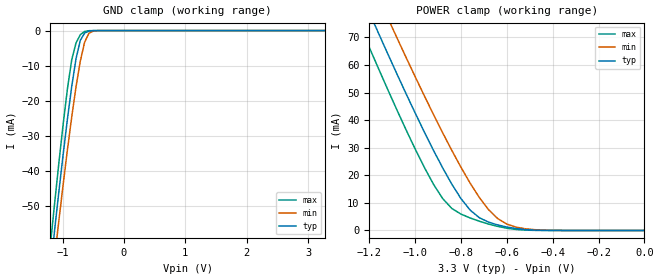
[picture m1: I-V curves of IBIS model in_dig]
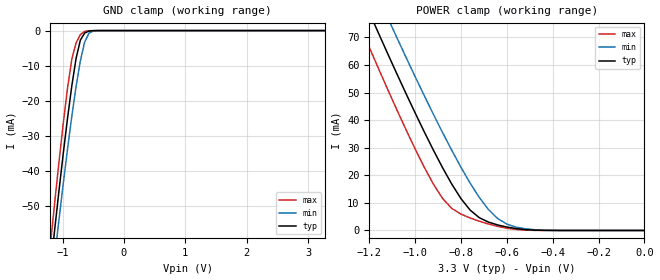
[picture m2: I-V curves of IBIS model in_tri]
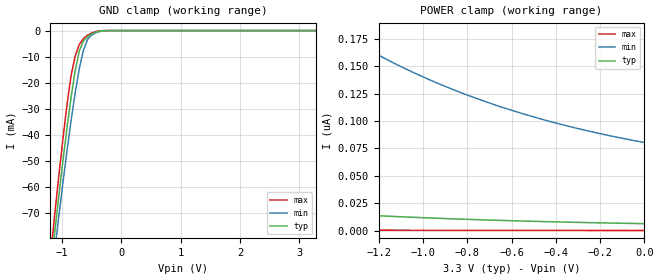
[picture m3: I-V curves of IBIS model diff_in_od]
| Integrated Devices Technolgy, Inc
[Ibis Ver]   4.1
[File Name]   9zxl1930d.ibs
[File Rev]   1.0
[Date]   Tuesday, January 30, 2018
[Source]   Integrated Devices Technolgy, Inc.
[Notes]   Rev 1.0 created by EvK
[Disclaimer] Integrated Device Technology, Inc. ("IDT") hereby grants the
   user of this IBIS model a non-exclusive, nontransferable
   license to use this IBIS model under the following terms. The
   user is granted this license only to use the IBIS model and is
   not granted rights to sell, copy (except as needed to run the
   IBIS model), rent, lease or sub-license the IBIS model in
   whole or in part, or in modified form to anyone. The User may
   modify the IBIS model to suit its specific applications, but
   rights to derivative works and such modifications shall belong
   to IDT. This IBIS model is provided on an AS IS" basis and IDT
   makes absolutely no warranty with respect to the information
   contained herein. IDT DISCLAIMS AND CUSTOMER WAIVES ALL
   WARRANTIES, EXPRESS AND IMPLIED, INCLUDING WARRANTIES OF
   MERCHANTABILITY AND FITNESS FOR A PARTICULAR PURPOSE. THE
   ENTIRE RISK AS TO QUALITY AND PERFORMANCE IS WITH THE USER
   ACCORDINGLY, IN NO EVENT SHALL IDT BE LIABLE FOR ANY DIRECT OR
   INDIRECT DAMAGES, WHETHER IN CONTRACT OR TORT, INCLUDING ANY
   LOST PROFITS OR OTHER INCIDENTAL, CONSEQUENTIAL, EXEMPLARY, OR
   PUNITIVE DAMAGES ARISING OUT OF THE USE OR APPLICATION OF THE
   IBIS model. Further, IDT reserves the right to make changes
   without notice to any product herein to improve reliability,
   function, or design. IDT does not convey any license under
   patent rights or any other intellectual property rights,
   including those of third parties. IDT is not obligated to
   provide maintenance or support for the licensed IBIS model.
   (C) Copyright Integrated Device Technology, Inc. 2016 All
   rights reserved
|   COMPONENT: ICS9zxl1930d
[Component]   ICS9zxl1930d
[Manufacturer]   Integrated Device Technology, Inc.
[Package]
| variable   typ   min   max
R_pkg   81.10m   62.20m   100.00m
L_pkg   6.70nH   4.90nH   8.50nH
C_pkg   0.53pF   0.21pF   0.85pF
[Pin]   signal_name   model_name   R_pin   L_pin   C_pin
1   VDDA   POWER
2   GNDA   GND
3   100M_133M#   in_dig
4   HBW_BYP_LBW#  in_tri
5   CKPWRGD_PD#   in_dig
6   GND   GND
7   VDDR   POWER
8   DIF_IN   diff_in_od
9   DIF_IN#   diff_in_od
10   SADR0_TRI   in_tri_od
11   SMBDAT   sda_od
12   SMBCLK   scl_od
13   SADR1_TRI   in_tri_od
14   FBOUT_NC#   NC
15   FBOUT_NC   NC
16   GND   GND
17   DIF_0   diff_out
18   DIF_0#   diff_out
19   DIF_1   diff_out
20   DIF_1#   diff_out
21   VDDIO   POWER
22   GND   GND
23   DIF_2   diff_out
24   DIF_2#   diff_out
25   DIF_3   diff_out
26   DIF_3#   diff_out
27   GND   GND
28   VDD   POWER
29   DIF_4   diff_out
30   DIF_4#   diff_out
31   DIF_5   diff_out
32   DIF_5#   diff_out
33   VDDIO   POWER
34   GND   GND
35   DIF_6   diff_out
36   DIF_6#   diff_out
37   DIF_7   diff_out
38   DIF_7#   diff_out
39   GND   GND
40   VDDIO   POWER
41   DIF_8   diff_out
42   DIF_8#   diff_out
43   DIF_9   diff_out
44   DIF_9#   diff_out
45   VDD   POWER
46   GND   GND
47   DIF_10   diff_out
48   DIF_10#   diff_out
49   DIF_11   diff_out
50   DIF_11#   diff_out
51   GND   GND
52   VDDIO   POWER
53   DIF_12   diff_out
54   DIF_12#   diff_out
55   DIF_13   diff_out
56   DIF_13#   diff_out
57   VDDIO   POWER
58   GND   GND
59   DIF_14   diff_out
60   DIF_14#   diff_out
61   DIF_15   diff_out
62   DIF_15#   diff_out
63   GND   GND
64   VDD   POWER
65   DIF_16   diff_out
66   DIF_16#   diff_out
67   DIF_17   diff_out
68   DIF_17#   diff_out
69   VDDIO   POWER
70   GND   GND
71   DIF_18   diff_out
72   DIF_18#   diff_out
73   EPAD   GND
[Diff Pin]   inv_pin   vdiff   tdelay_typ
8   9   NA   NA
15   14   NA   NA
17   18   NA   NA
19   20   NA   NA
23   24   NA   NA
25   26   NA   NA
29   30   NA   NA
31   32   NA   NA
35   36   NA   NA
37   38   NA   NA
41   42   NA   NA
43   44   NA   NA
47   48   NA   NA
49   50   NA   NA
53   54   NA   NA
55   56   NA   NA
59   60   NA   NA
61   62   NA   NA
65   66   NA   NA
67   68   NA   NA
71   72   NA   NA
[Model Selector] diff_out
clk_out   HCSL Diff output enabled
hcsl_hiz   HCSL Diff output disabled to Hi-Z
| Models and submodels in the file (8): in_dig (Input), in_tri (Input), diff_in_od (Input), in_tri_od (Input), sda_od (I/O_open_drain), scl_od (Input), hcsl_hiz (Input), clk_out (Output)
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|   Model in_dig
[Model]  in_dig
Model_type Input
Polarity   Non-Inverting
Vinl =   0.8000V
Vinh =   2.0000V
C_comp   2.1000pF   2.1000pF   2.1000pF
[Temperature Range]   25.0000   85.0000   -40.0000
[Voltage Range]   3.3000V   3.1350V   3.4650V
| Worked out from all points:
|   GND clamp passes 1 mA (typ) near -0.65 V on its own axis
|   POWER clamp passes 1 mA (typ) near -0.58 V on its own axis
[GND_clamp]
|Voltage   I(typ)   I(min)   I(max)
-3.3V     -444.4mA   -436.3mA   -455.2mA
-1.2V     -68.37mA   -75.7mA    -61.37mA
-1.13V    -56.99mA   -64.8mA    -49.35mA
-1.06V    -45.92mA   -54.16mA   -37.72mA
-920mV    -25.14mA   -33.91mA   -16.51mA
-850mV    -15.84mA   -24.53mA   -8.255mA
-780mV    -7.95mA    -15.96mA   -3.499mA
-710mV    -2.728mA   -8.626mA   -1.156mA
-640mV    -697.7uA   -3.286mA   -240.6uA
-570mV    -146.6uA   -751uA     -34.01uA
-430mV    -3.844uA   -23.08uA   -279.3nA
3.28V     213.4pA    44.16nA    205.9pA
[POWER_clamp]
|Voltage   I(typ)   I(min)   I(max)
-3.28V    509.3mA    515.8mA    504.9mA
-1.24V    86.61mA    99.33mA    74.1mA
-1.16V    71.55mA    84.5mA     58.72mA
-1.12V    64.14mA    77.19mA    51.18mA
-1.08V    56.84mA    69.96mA    43.78mA
-960mV    35.71mA    48.84mA    22.88mA
-880mV    22.69mA    35.43mA    11.57mA
-840mV    16.77mA    29.02mA    7.979mA
-760mV    7.367mA    17.14mA    4.53mA
-640mV    2.005mA    4.321mA    1.477mA
-480mV    131.2uA    293.3uA    37.64uA
0V        220.8pA    394.5pA    228.5pA
|   Model in_tri
[Model]  in_tri
Model_type Input
Polarity   Non-Inverting
Vinl =   0.8000V
Vinh =   2.0000V
C_comp   2.1400pF   2.1400pF   2.1400pF
[Temperature Range]   25.0000   85.0000   -40.0000
[Voltage Range]   3.3000V   3.1350V   3.4650V
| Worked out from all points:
|   GND clamp passes 1 mA (typ) near -0.65 V on its own axis
|   POWER clamp passes 1 mA (typ) near -0.58 V on its own axis
[GND_clamp]
|Voltage   I(typ)   I(min)   I(max)
-3.3V     -444.4mA   -436.3mA   -455.2mA
-1.2V     -68.37mA   -75.7mA    -61.37mA
-1.13V    -56.99mA   -64.8mA    -49.35mA
-1.06V    -45.92mA   -54.16mA   -37.72mA
-920mV    -25.14mA   -33.91mA   -16.51mA
-850mV    -15.84mA   -24.53mA   -8.255mA
-780mV    -7.95mA    -15.96mA   -3.499mA
-710mV    -2.728mA   -8.625mA   -1.156mA
-640mV    -697.7uA   -3.286mA   -240.6uA
-570mV    -146.6uA   -751uA     -34.01uA
-430mV    -3.844uA   -23.08uA   -279.3nA
3.28V     213.4pA    44.16nA    205.9pA
[POWER_clamp]
|Voltage   I(typ)   I(min)   I(max)
-3.28V    509.3mA    515.8mA    504.9mA
-1.24V    86.61mA    99.33mA    74.1mA
-1.16V    71.55mA    84.5mA     58.72mA
-1.12V    64.14mA    77.19mA    51.18mA
-1.08V    56.84mA    69.96mA    43.78mA
-960mV    35.71mA    48.84mA    22.88mA
-880mV    22.69mA    35.43mA    11.57mA
-840mV    16.77mA    29.02mA    7.979mA
-760mV    7.367mA    17.14mA    4.53mA
-640mV    2.005mA    4.321mA    1.477mA
-480mV    131.2uA    293.3uA    37.64uA
0V        220.8pA    394.5pA    228.4pA
|   Model diff_in_od
[Model]  diff_in_od
Model_type Input
Polarity   Non-Inverting
Vinl =   0.3000V
Vinh =   0.5000V
C_comp   3.5000pF   3.5000pF   3.5000pF
[Temperature Range]   25.0000   85.0000   -40.0000
[Voltage Range]   3.3000V   3.1350V   3.4650V
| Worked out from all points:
|   GND clamp passes 1 mA (typ) near -0.47 V on its own axis
[GND_clamp]
|Voltage   I(typ)   I(min)   I(max)
-3.3V     -581.4mA   -566.8mA   -600.3mA
-1.2V     -92.9mA    -99.3mA    -87.17mA
-1.13V    -78.34mA   -85.45mA   -71.6mA
-1.06V    -64.19mA   -71.96mA   -56.52mA
-920mV    -37.64mA   -46.39mA   -28.76mA
-850mV    -25.69mA   -34.6mA    -17.37mA
-780mV    -15.32mA   -23.82mA   -9.726mA
-710mV    -7.779mA   -14.52mA   -5.31mA
-640mV    -3.984mA   -7.427mA   -3.004mA
-500mV    -1.282mA   -1.675mA   -939.5uA
-220mV    -3.662uA   -14.35uA   -357.2nA
3.28V     6.54nA     86.14nA    391.5pA
[POWER_clamp]
|Voltage   I(typ)   I(min)   I(max)
-3.28V    57.48nA    654.6nA    1.522nA
-2.84V    43.19nA    492.3nA    1.256nA
-2.4V     32.05nA    365.8nA    1.04nA
-1.92V    22.9nA     262.2nA    852pA
-1.4V     15.85nA    182.8nA    693.7pA
-1.12V    13.05nA    151.5nA    623.8pA
-960mV    11.71nA    136.6nA    587.9pA
-800mV    10.54nA    123.6nA    554.6pA
-640mV    9.52nA     112.3nA    523.5pA
-440mV    8.427nA    100.3nA    487.7pA
-240mV    7.511nA    90.3nA     454.6pA
0V        6.607nA    80.43nA    417.9pA
